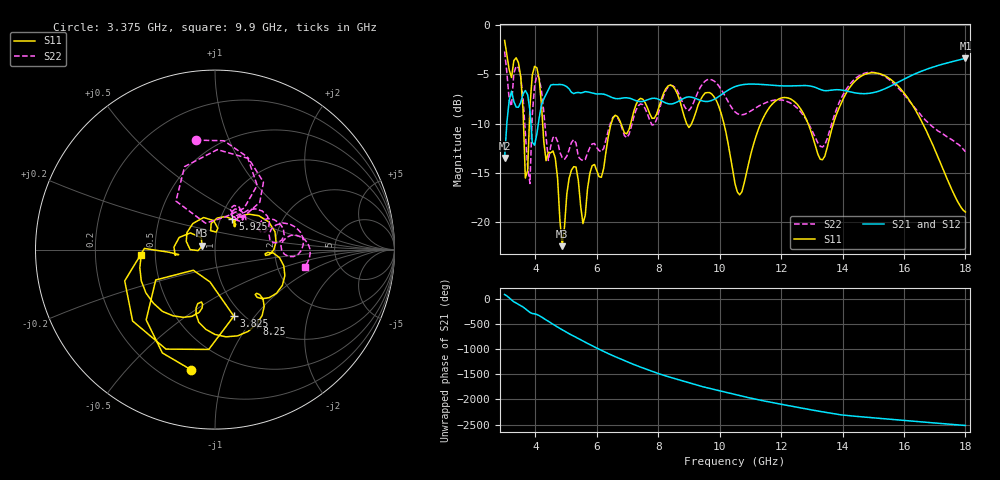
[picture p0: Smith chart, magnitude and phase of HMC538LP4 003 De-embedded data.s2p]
! Chelmsford, MA 01824
! http://www.hittite.com
! Tel: 978-250-3343
! Fax: 978-250-3373
! Device  :  HMC538LP4
! Description:  600 Analog Phase Shifter
! Frequency  :  6.0 GHz - 15.0 GHz
! Package  :  LP4  - 4x4 mm Quad Flatpack No-Lead (QFN) Plastic Package: 24 pin
! Ports  :  2 RF, 1 DC
!  Pin  3  = Rfin  = Port 1
!  Pin  16  = Rfout = Port 2
!  pin  21  = vCTL
! Voltages:  VCTL  = 0 to 5.0 Volts
! Currents :  Vb(V)  Vd(V)  Ib(mA)  Id(mA)
!  0.00  0.30  0.000000	0.486057
! Data:  The device was measured on evaluation board 111296-1.
!  Data was collected using a calibrated network analyzer.
!  The evaluation circuit board was modeled and simulated.This was use
!  to removed the evaluation board circuit from the measured data.
!  The reference plane is the center of the package pin.
! Misc:  Lot #
!Date Measured:  03 - 11 -2009
! Date:  03 - 17 -2009
! Note:
!  Hittite Microwave supplies this data as a sample of measured data at the
!  package pin for this package product.  Your particular data for this product
!  may vary.
!  Data was taken at 25 degrees C.
!  Hittite Microwave reserves the right to change this data at anytime.
# MHz S MA R 50
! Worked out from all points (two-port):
!   201 points, 3 GHz to 18 GHz, reference 50 ohm
!   highest |S21| = -3.36 dB at 18 GHz (marker M1); lowest = -13.5 dB at 3 GHz (marker M2)
!   |S21| within 3 dB of the highest: 10.42 GHz to 13.15 GHz (2.727 GHz wide, 23.1 % of centre); 15.45 GHz to end of sweep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
!   lowest |S11| = -22.5 dB at 4.875 GHz (marker M3), VSWR 1.16, Z = 43.3 + j1.86 ohm
!   |S11| at or under -10 dB: 4.238 GHz to 6.47 GHz (2.232 GHz wide, 41.7 % of centre); 10.14 GHz to 11.34 GHz (1.2 GHz wide, 11.2 % of centre); 16.61 GHz to end of sweep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
!   |S22| runs from -16.1 to -2.7 dB; largest |S21 - S12| = 0.0018
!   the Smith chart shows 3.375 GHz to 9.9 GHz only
!   S11 on the Smith chart (normalised r, x): 3.375 GHz: 0.31, -0.78; 3.825 GHz: 0.91, -0.79; 5.925 GHz: 1.14, +0.40; 8.25 GHz: 1.01, -1.09; 9.9 GHz: 0.42, -0.03
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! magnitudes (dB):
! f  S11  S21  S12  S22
! 3 GHz  -1.5  -13.5  -13.5  -2.7
! 3.225 GHz  -5.3  -6.7  -6.7  -8.2
! 3.375 GHz  -3.3  -8.3  -8.3  -4.2
! 3.525 GHz  -5.2  -7.8  -7.9  -5.2
! 3.675 GHz  -15.6  -6.6  -6.6  -11.0
! 3.825 GHz  -8.3  -8.7  -8.7  -16.1
! 4.05 GHz  -4.3  -11.1  -11.1  -5.1
! 4.425 GHz  -12.9  -6.6  -6.6  -13.8
! 4.65 GHz  -13.5  -6.0  -6.0  -11.3
! 4.875 GHz  -22.5  -6.0  -6.1  -13.5
! 5.25 GHz  -14.4  -6.9  -7.0  -11.6
! 5.55 GHz  -20.2  -6.8  -6.8  -13.8
! 5.925 GHz  -14.2  -6.9  -7.0  -12.0
! 8.025 GHz  -8.3  -7.6  -7.6  -8.8
! 8.25 GHz  -6.4  -7.9  -7.9  -6.6
! 9 GHz  -10.4  -7.3  -7.3  -8.7
! 9.9 GHz  -7.7  -7.4  -7.4  -5.9
! 10.5 GHz  -16.1  -6.2  -6.2  -8.8
! 11.93 GHz  -7.5  -6.1  -6.2  -7.6
! 13.05 GHz  -11.6  -6.3  -6.3  -11.0
! 15.53 GHz  -5.4  -6.2  -6.3  -5.5
! 18 GHz  -19.0  -3.4  -3.4  -12.9
